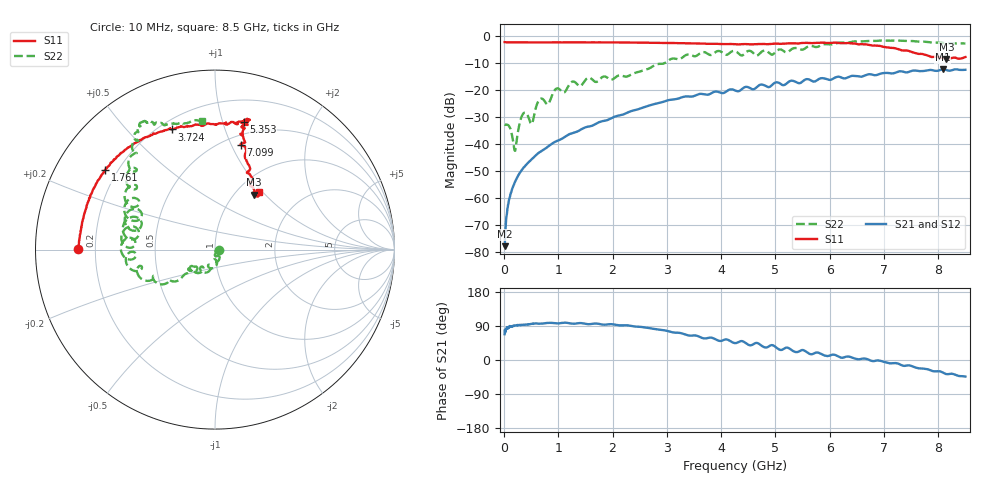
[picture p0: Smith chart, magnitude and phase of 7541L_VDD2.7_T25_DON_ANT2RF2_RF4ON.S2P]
!Agilent Technologies,E5071C,MY46417908,A.11.23
!Date: Wed Dec 09 17:18:22 2020
!Data & Calibration Information:
!Freq	S11:SOLT2(ON)	S21:SOLT2(ON)	S12:SOLT2(ON)	S22:SOLT2(ON)
!PortZ  Port1:50+j0  Port2:50+j0
!Above PortZ is port z conversion or system Z0 setting when saving the data.
!When reading, reference impedance value at option line is always used.
# Hz S dB R 50
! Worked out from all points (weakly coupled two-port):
!   1601 points, 10 MHz to 8.5 GHz, reference 50 ohm
!   highest |S21| = -12.37 dB at 8.086 GHz (marker M1); lowest = -77.7 dB at 10 MHz (marker M2)
!   lowest |S11| = -8.5 dB at 8.15 GHz (marker M3), VSWR 2.20, Z = 60.8 + j43.2 ohm
!   |S11| at or under -10 dB: nowhere
!   |S22| runs from -42.5 to -1.7 dB; largest |S21 - S12| = 0.0022
!   S11 on the Smith chart (normalised r, x): 10 MHz: 0.13, +0.00; 1.761 GHz: 0.15, +0.32; 3.724 GHz: 0.25, +0.67; 5.353 GHz: 0.39, +1.17; 7.099 GHz: 0.59, +1.09; 8.5 GHz: 1.24, +0.96
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1e7  -2.33 179.7  -77.70 68.1  -76.96 84.6  -32.78 -6.9
8.42875e7  -2.39 178.0  -61.31 86.6  -61.58 86.7  -33.14 -48.9
2.01025e8  -2.41 175.4  -53.96 90.6  -53.99 91.2  -42.48 -46.5
3.230688e8  -2.44 172.6  -49.73 92.2  -49.72 92.7  -29.85 -45.6
3.973562e8  -2.44 171.0  -47.82 93.5  -47.84 93.4  -28.40 -78.5
5.034812e8  -2.44 168.6  -45.71 95.3  -45.74 95.2  -32.62 -76.7
6.626688e8  -2.44 165.3  -42.91 95.9  -42.90 95.9  -23.34 -79.7
8.059375e8  -2.45 162.4  -40.97 97.9  -40.97 97.9  -25.33 -91.1
9.65125e8  -2.43 159.1  -38.91 96.8  -38.91 96.8  -19.49 -99.4
1.426769e9  -2.42 150.1  -34.49 97.3  -34.50 97.3  -18.28 -121.8
1.761062e9  -2.44 144.1  -31.82 94.9  -31.81 95.1  -16.09 -131.5
2.843538e9  -2.61 126.2  -24.85 80.1  -24.86 80.2  -10.40 -145.3
3.724375e9  -2.96 109.7  -21.76 57.2  -21.77 57.2  -6.30 -177.4
4.255e9  -3.09 96.6  -20.17 44.6  -20.17 44.5  -5.62 169.3
4.658275e9  -3.08 88.6  -18.90 45.0  -18.92 44.9  -7.30 162.5
5.353394e9  -2.75 77.3  -16.83 21.8  -16.80 21.7  -4.51 146.6
5.671769e9  -2.71 76.0  -16.68 15.2  -16.62 15.2  -3.77 135.7
7.088538e9  -4.38 76.4  -13.76 -8.3  -13.79 -8.5  -1.85 119.8
7.09915e9  -4.42 76.2  -13.80 -8.6  -13.85 -8.7  -1.85 119.9
8.086112e9  -8.25 54.7  -12.37 -33.3  -12.38 -33.3  -2.68 107.4
8.149788e9  -8.53 54.7  -12.65 -37.2  -12.67 -37.1  -2.73 105.5
8.5e9  -7.84 52.8  -12.55 -43.7  -12.62 -43.7  -2.84 95.8
